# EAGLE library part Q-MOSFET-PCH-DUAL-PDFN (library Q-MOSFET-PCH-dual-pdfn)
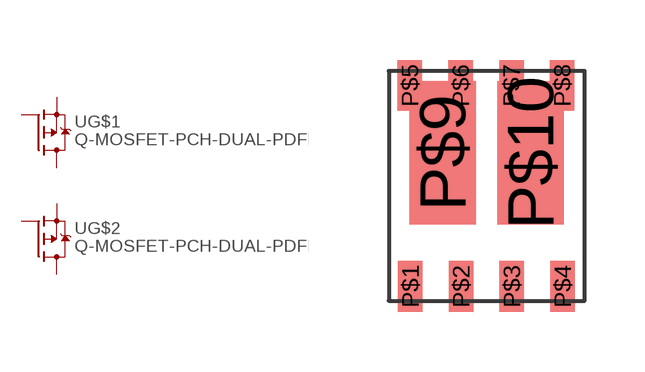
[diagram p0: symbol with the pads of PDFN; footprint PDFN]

Designator prefix -; gates G$1=P-MOSFET G$2=P-MOSFET

## Q-MOSFET-PCH-DUAL-PDFN  [PDFN]
P$1  G$1:S  pas
P$2  G$1:G  pas
P$3  G$2:S  pas
P$4  G$2:G  pas
P$5  G$1:D  pas
P$6  G$1:D  pas
P$7  G$2:D  pas
P$8  G$2:D  pas
P$9  G$1:D  pas
P$10  G$2:D  pas

## Footprint PDFN (pad centres in mm)
smd 0.61 x 1.27: P$1 -1.873,-2.688; P$2 -0.603,-2.688; P$3 0.667,-2.688; P$4 1.937,-2.688; P$5 -1.883,2.342; P$6 -0.613,2.342; P$7 0.657,2.342; P$8 1.927,2.342
smd 1.66 x 3.58: P$9 -1.063,0.652; P$10 1.137,0.652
